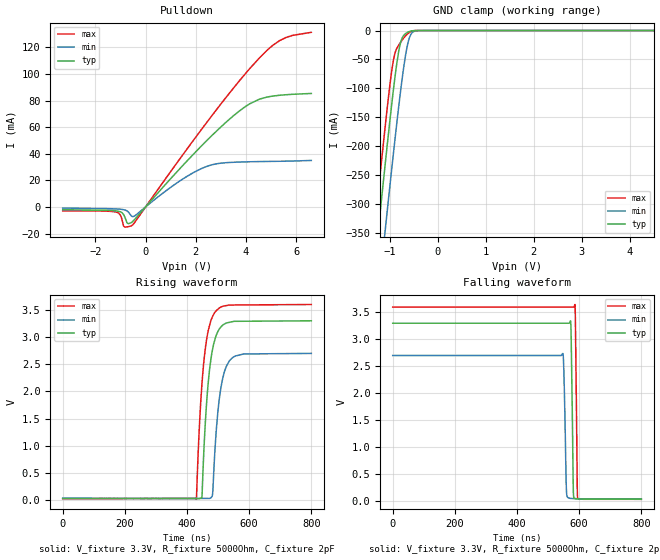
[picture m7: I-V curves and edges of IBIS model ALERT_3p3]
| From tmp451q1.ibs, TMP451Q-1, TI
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|   Model
[Model]   ALERT_3p3
Model_type   Open_drain
Polarity   Non-Inverting
Vmeas = 1.65
Vref = 3.3
Cref = 2pF
Rref = 5000
|   typ   min   max
C_comp   1.58pF   1.53pF   1.65pF
[Voltage Range]   3.3   2.7   3.6
[Temperature Range]   25   125   -40
[Pullup Reference]   3.3   2.7   3.6
[Pulldown Reference]   -0   0   -0
[Power Clamp Reference]   3.3   2.7   3.6
[GND Clamp Reference]   0   0   0
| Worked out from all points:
|   slope of the pulldown table from 0 to 0.495 V, typ, clamps not added: 46.6 ohm
|   GND clamp passes 1 mA (typ) near -0.56 V on its own axis
|   falling waveform, V_fixture 3.3V, R_fixture 5000Ohm, C_fixture 2pF: 20-80 % time 4.66ns typ, 5.58ns min, 4.16ns max; typ from 3.3 V to 0.03 V
|   rising waveform, V_fixture 3.3V, R_fixture 5000Ohm, C_fixture 2pF: 20-80 % time 25.8ns typ, 25.8ns min, 26.2ns max; typ from 0.03 V to 3.3 V
[Pulldown]
|   Voltage   I(typ)   I(min)   I(max)
-3.3V     -2.101mA   -839.5uA   -2.905mA
-1.171V   -2.97mA    -1.491mA   -3.848mA
-993.3mV  -3.716mA   -1.732mA   -6.477mA
-874.5mV  -5.682mA   -2.04mA    -14.45mA
-716.1mV  -12.32mA   -3.283mA   -14.9mA
-537.9mV  -11.33mA   -7.13mA    -13.84mA
2.095V    43.35mA    27.68mA    54.95mA
2.788V    56.38mA    32.31mA    72.27mA
3.897V    74.41mA    33.85mA    98.47mA
4.531V    80.99mA    34.11mA    112mA
5.333V    83.94mA    34.34mA    125mA
6.6V      85.32mA    34.96mA    131.3mA
[GND Clamp]
|   Voltage   I(typ)   I(min)   I(max)
-3.3V     -2.079A    -2.184A    -2.022A
-1.379V   -459mA     -573.7mA   -393.2mA
-1.211V   -322mA     -437mA     -255.9mA
-1.102V   -235.3mA   -349.9mA   -169.8mA
-943.8mV  -115.1mA   -226.5mA   -60.21mA
-884.4mV  -74.64mA   -181.7mA   -36.69mA
-815.1mV  -35.74mA   -131.4mA   -25.18mA
-735.9mV  -11.75mA   -78.51mA   -15.56mA
-607.2mV  -2.215mA   -16.42mA   -4.165mA
-528mV    -454.6uA   -3.149mA   -798.7uA
-399.3mV  -8.342uA   -116uA     -5.561uA
6.6V      0A         0A         0A
[Ramp]
R_load = 5000
|   typ   min   max
dV/dt_r   1.96189/2.57804e-08   1.59959/2.56669e-08   2.14406/2.62339e-08
dV/dt_f   1.96189/4.65834e-09   1.59959/5.57765e-09   2.14406/4.15991e-09
[Falling Waveform]
V_fixture = 3.3V
V_fixture_min = 2.7V
V_fixture_max = 3.6V
R_fixture = 5000Ohm
C_fixture = 2pF
|   Time   V(typ)   V(min)   V(max)
0s        3.3V       2.7V       3.6V
547.4ns   3.3V       2.737V     3.6V
551ns     3.3V       2.347V     3.6V
559ns     3.3V       194.9mV    3.6V
572ns     3.345V     44.07mV    3.6V
574.6ns   2.893V     42.88mV    3.6V
581.1ns   213.9mV    39.92mV    3.6V
586.4ns   43.61mV    37.51mV    3.648V
595.3ns   34.83mV    36.51mV    45.3mV
800ns     30.19mV    34mV       26.56mV
[Rising Waveform]
V_fixture = 3.3V
V_fixture_min = 2.7V
V_fixture_max = 3.6V
R_fixture = 5000Ohm
C_fixture = 2pF
|   Time   V(typ)   V(min)   V(max)
0s        30.19mV    34mV       26.56mV
430.2ns   27.24mV    31.42mV    14.35mV
447.8ns   42.58mV    31.32mV    2.118V
453ns     757.3mV    31.29mV    2.483V
467.3ns   2.101V     31.2mV     3.091V
481.7ns   2.76V      89.77mV    3.372V
486.1ns   2.879V     516mV      3.424V
507ns     3.173V     1.994V     3.547V
537.2ns   3.273V     2.569V     3.59V
800ns     3.3V       2.7V       3.6V
